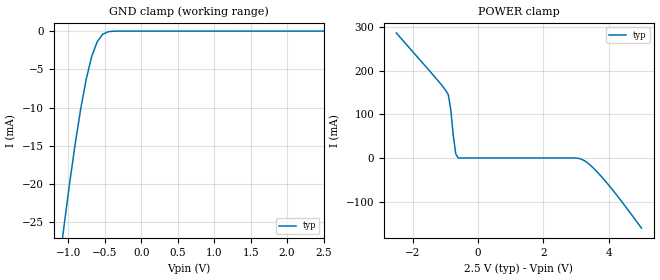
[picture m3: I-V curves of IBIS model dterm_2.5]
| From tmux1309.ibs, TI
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| dterm_2.5
[Model]   dterm_2.5
Model_type   Terminator
|   typ   min   max
C_comp   4.014581e-12   NA   NA
[Voltage Range]   2.5   NA   NA
[Temperature Range]   27   NA   NA
[Power Clamp Reference]   2.5   NA   NA
[GND Clamp Reference]   0   NA   NA
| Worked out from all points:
|   GND clamp passes 1 mA (typ) near -0.57 V on its own axis
|   POWER clamp passes 1 mA (typ) near -0.61 V on its own axis
[GND Clamp]
|   Voltage   I(typ)   I(min)   I(max)
-5V       -20.06kA   NA         NA
-1.136V   -31.34mA   NA         NA
-1.061V   -25.5mA    NA         NA
-984.8mV  -19.99mA   NA         NA
-909.1mV  -14.88mA   NA         NA
-833.3mV  -10.29mA   NA         NA
-757.6mV  -6.376mA   NA         NA
-681.8mV  -3.367mA   NA         NA
-606.1mV  -1.403mA   NA         NA
-530.3mV  -420.5uA   NA         NA
-303mV    -1.846uA   NA         NA
2.5V      620.2pA    NA         NA
[POWER Clamp]
|   Voltage   I(typ)   I(min)   I(max)
-2.5V     287.4mA    NA         NA
-1.212V   176.6mA    NA         NA
-909.1mV  145.3mA    NA         NA
-833.3mV  111.2mA    NA         NA
-757.6mV  52.94mA    NA         NA
-681.8mV  9.727mA    NA         NA
-606.1mV  26.88uA    NA         NA
2.879V    -14.65uA   NA         NA
3.182V    -3.367mA   NA         NA
3.485V    -19.99mA   NA         NA
3.864V    -50.35mA   NA         NA
5V        -161.2mA   NA         NA
